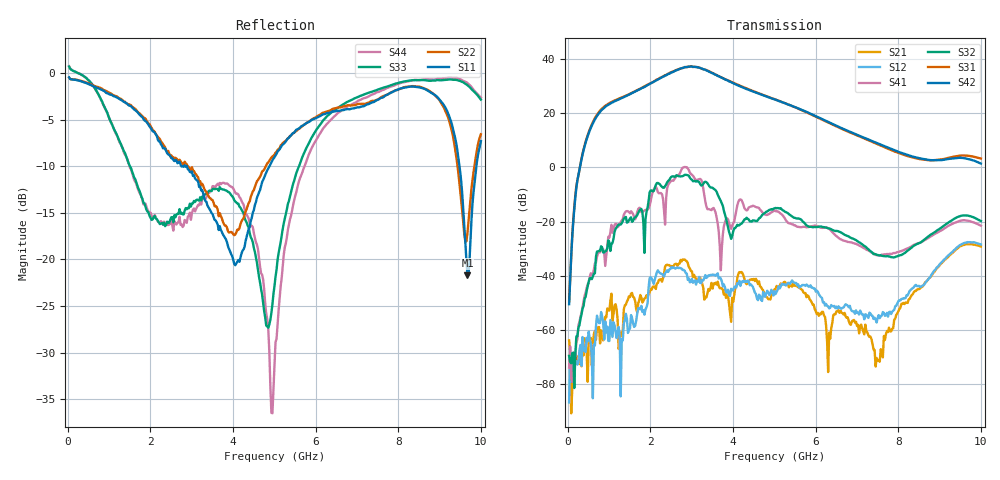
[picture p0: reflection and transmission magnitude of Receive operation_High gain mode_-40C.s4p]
! Device:  ADRF5545A
! Description: Dual-Channel, Receiver Front End
! Frequency:  2.4 -  4.2 GHz
! Ports:
!	ANT-CHA	= Port 1
!	ANT-CHB	= Port 2
!  RXOUT-CHA = Port 3
!	RXOUT-CHB = Port 4
! VDD1-CHA, VDD1-CHB, VDD2-CHA, VDD2-CHB, and SWVDD-CHAB = 5 V
! SWCTRL-CHAB = 0 V,  PD-CHAB = 0 V,BP-CHA=BP-CHB=0V
! Temp=-40C
! Data:  Data was collected using a calibrated 4 port network analyzer and de-embedded using AtaiTec's In Situ De-Embedding.
! Note:  Analog Devices supplies this data as a sample of measured data
!  for this product.  Your particular data for this product may vary.
!  Data was taken at -40 degrees C.
!  Analog Devices reserves the right to change this data at anytime.
!Correction: S11(Full 4 Port(1,2,3,4))
!S12(Full 4 Port(1,2,3,4))
!S13(Full 4 Port(1,2,3,4))
!S14(Full 4 Port(1,2,3,4))
!S21(Full 4 Port(1,2,3,4))
!S22(Full 4 Port(1,2,3,4))
!S23(Full 4 Port(1,2,3,4))
!S24(Full 4 Port(1,2,3,4))
!S31(Full 4 Port(1,2,3,4))
!S32(Full 4 Port(1,2,3,4))
!S33(Full 4 Port(1,2,3,4))
!S34(Full 4 Port(1,2,3,4))
!S41(Full 4 Port(1,2,3,4))
!S42(Full 4 Port(1,2,3,4))
!S43(Full 4 Port(1,2,3,4))
!S44(Full 4 Port(1,2,3,4))
!S4P File: Measurements: <S11,S12,S13,S14>,
!<S21,S22,S23,S24>,
!<S31,S32,S33,S34>,
!<S41,S42,S43,S44>:
# Hz S  dB  R 50
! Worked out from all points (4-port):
!   400 points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, 34.98 MHz to 10 GHz, reference 50 ohm
!   strongest paths, dB at 34.98 MHz, 2.532 GHz, 5.03 GHz, 7.527 GHz, 10 GHz:
!     S42: -50.4, 35.1, 24.9, 8.7, 1.4
!     S31: -49.3, 35.3, 25.0, 8.4, 3.2
!     S32: -69.5, -3.3, -15.0, -32.4, -19.8
!     S41: -73.8, -4.9, -16.2, -32.4, -21.5
!     S12: -86.6, -37.1, -46.7, -54.5, -28.4
!     S21: -63.8, -36.7, -44.9, -71.0, -29.2
!   lowest |S11| = -21.7 dB at 9.675 GHz (marker M1), VSWR 1.18, Z = 44.9 + j5.85 ohm
!   |S11| at or under -10 dB: 2.752 GHz to 2.816 GHz (63.69 MHz wide, 2.29 % of centre); 2.884 GHz to 4.883 GHz (1.999 GHz wide, 51.5 % of centre); 9.482 GHz to 9.892 GHz (409.8 MHz wide, 4.23 % of centre)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
3.4975e7  -0.46 -11.3  -86.64 -7.1  -75.20 -142.1  -67.25 -173.5
          -63.78 69.8  -0.49 -11.1  -68.55 109.9  -62.10 -145.7
          -49.34 -76.3  -69.50 -46.8  0.69 -10.5  -65.10 27.9
          -73.84 153.9  -50.42 -96.0  -65.18 35.3  0.74 -10.4
1.833175e9  -4.93 -126.6  -52.70 -168.1  -60.65 93.7  -79.83 -86.1
            -49.28 -174.4  -4.76 -130.8  -71.78 106.4  -63.07 81.2
            29.65 -46.0  -20.69 -86.2  -13.93 145.7  -48.09 -97.6
            -16.18 -52.9  29.48 -46.3  -47.87 -136.3  -14.11 144.4
2.882125e9  -9.97 84.1  -39.18 33.2  -57.41 39.4  -85.64 -87.7
            -34.59 26.0  -9.79 83.6  -75.58 67.8  -57.91 31.4
            37.08 173.4  -2.79 78.4  -14.62 13.3  -46.96 152.4
            0.08 84.7  36.92 173.5  -51.01 36.2  -16.07 12.2
3.25675e9  -12.55 12.2  -41.47 36.6  -57.46 16.3  -70.91 39.0
           -42.86 -22.4  -11.88 11.5  -72.72 91.0  -59.22 -0.6
           36.31 111.8  -6.59 -12.8  -13.27 -15.5  -51.51 136.2
           -5.54 -48.5  36.39 109.5  -47.38 112.1  -13.47 -25.9
3.881125e9  -18.60 -45.4  -45.11 -16.0  -59.06 -16.5  -69.54 64.8
            -47.27 -8.6  -17.00 -29.0  -76.60 100.0  -58.21 -8.8
            32.08 31.4  -22.34 88.4  -12.76 -39.4  -46.93 117.2
            -19.15 -129.2  31.96 29.3  -46.18 83.4  -11.93 -44.6
9.675325e9  -21.73 127.8  -27.54 -132.1  -59.82 34.2  -61.33 21.7
            -28.37 -138.7  -17.15 143.4  -62.87 -43.5  -70.92 61.6
            4.32 -27.1  -17.75 -92.8  -1.31 89.7  -57.79 73.2
            -19.64 -79.8  3.17 -38.9  -63.44 52.4  -1.07 85.4
1e10  -7.31 -156.9  -28.41 168.9  -63.45 72.2  -64.95 17.0
      -29.16 165.9  -6.57 173.1  -69.06 -61.2  -64.88 74.1
      3.25 -66.1  -19.77 -153.5  -2.85 89.5  -57.54 75.3
      -21.50 -137.3  1.41 -75.8  -69.87 -26.7  -2.63 86.2
